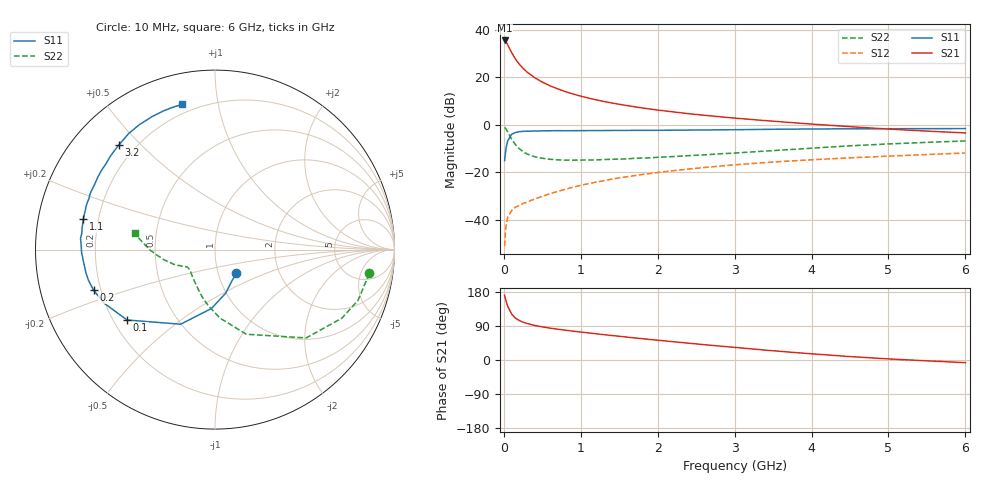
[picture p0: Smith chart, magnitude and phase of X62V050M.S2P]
! SIEMENS Small Signal Semiconductors
! BFP193W
! Si NPN RF Bipolar Junction Transistor in SOT343
! VCE = 2 V  IC = 50 mA
! Common Emitter S-Parameters:  April 1994
# GHz  S  MA  R  50
!  f  S11  S21  S12  S22
! GHz  MAG  ANG  MAG  ANG  MAG  ANG  MAG  ANG
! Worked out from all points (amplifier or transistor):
!   40 points, 10 MHz to 6 GHz, reference 50 ohm
!   highest |S21| = 35.4 dB at 10 MHz (marker M1)
!   |S21| within 3 dB of that: start of sweep to 68.39 MHz
!   unconditionally stable (mu >= 1): 500.5 MHz to 4.338 GHz
!   at 200 MHz: K = 0.63, MSG = 29.7 dB, |S12| = -34.0 dB
!   at 1.5 GHz: K = 1.16, MAG = 13.0 dB, |S12| = -22.3 dB
!   at 6 GHz: K = 0.96, MSG = 4.2 dB, |S12| = -11.9 dB
!   S11 on the Smith chart (normalised r, x): 10 MHz: 1.21, -0.33; 100 MHz: 0.26, -0.33; 200 MHz: 0.17, -0.16; 1.1 GHz: 0.14, +0.11; 3.2 GHz: 0.14, +0.43; 6 GHz: 0.15, +0.79
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0.01  0.1764 -49.0  59.07 170.6  0.0028 83.1  0.87 -8.8
0.02  0.2509 -76.5  57.41 162.9  0.0055 72.8  0.8456 -19.5
0.03  0.3284 -93.4  54.86 155.1  0.0077 70.9  0.8036 -28.4
0.05  0.4575 -114.7  47.88 141.9  0.0114 60.3  0.7072 -44.1
0.1  0.6275 -141.3  33.12 121.7  0.0157 47.2  0.5029 -69.7
0.15  0.6862 -154.2  24.2 110.6  0.0185 44.0  0.3823 -85.9
0.2  0.7134 -161.5  18.79 104.2  0.02 44.4  0.3133 -97.1
0.25  0.7257 -166.5  15.36 99.8  0.0221 46.7  0.2724 -105.3
0.3  0.7308 -170.0  12.86 96.5  0.0236 49.0  0.2429 -112.2
0.4  0.7368 -175.3  9.763 91.3  0.0275 52.7  0.2125 -122.0
0.5  0.7436 -178.9  7.868 87.4  0.0312 55.3  0.1972 -129.1
0.6  0.7463 177.9  6.573 84.1  0.0355 57.7  0.1879 -134.5
0.8  0.7475 173.0  4.964 78.6  0.0441 60.8  0.18 -140.8
1  0.7509 169.0  3.977 73.8  0.0533 62.5  0.1809 -145.2
1.1  0.753 167.0  3.639 71.5  0.0578 62.9  0.1808 -146.5
1.3  0.755 163.0  3.085 66.9  0.0666 63.0  0.1851 -148.3
1.6  0.7576 157.8  2.529 60.4  0.0807 62.5  0.1916 -150.4
2.2  0.7681 148.0  1.862 48.3  0.1081 59.5  0.2142 -155.5
3.2  0.792 132.4  1.297 29.7  0.1516 52.3  0.2667 -164.7
4.5  0.8196 115.4  0.91 9.0  0.2014 42.2  0.3604 -179.4
5.5  0.8268 106.9  0.734 -2.2  0.2363 35.3  0.4261 171.9
6  0.8301 102.8  0.672 -7.0  0.2545 32.2  0.456 168.5
